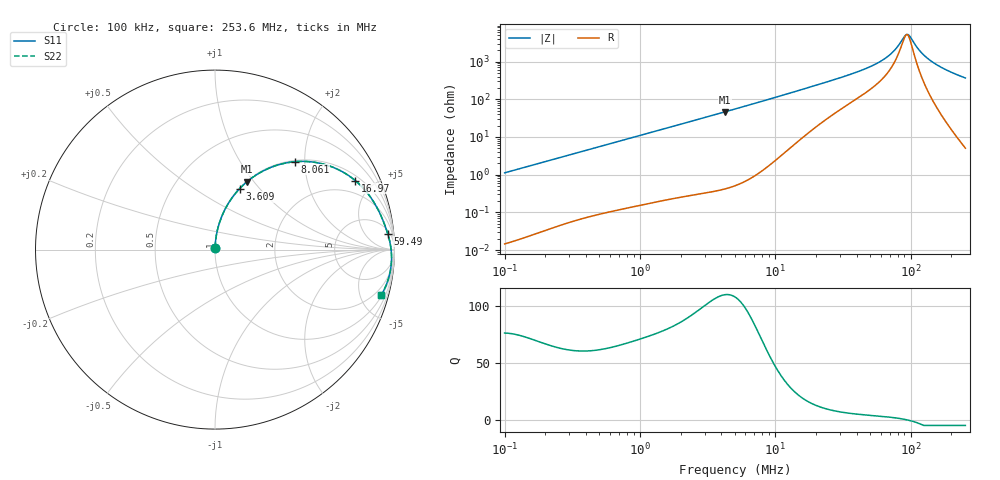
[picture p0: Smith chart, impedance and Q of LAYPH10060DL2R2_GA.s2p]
! LAYPH10060DL2R2_GA  S-PARAMETER MODEL  ( General Type )
! Model Generated by TAIYO YUDEN Corporation (http://www.ty-top.com)
! Version 3.0
! TAIYO YUDEN Control No. 180828NI43SB-FBB
! Copyright(c) 2017 TAIYO YUDEN CO.,LTD. All Rights Reserved.
! Product Description (link to TY-COMPAS)
! https://ds.yuden.co.jp/TYCOMPAS/or/detail?pn=LAYPH10060DL2R2NGA&u=M
! Products Name : Inductors
! Characteristics :
!  Inductance : 2.2 uH , SRF(min) : -Hz , DC Resistance(max) : 0.009 Ohm
!  Rated Current : Saturation :7.5 A , Temp Rise : 5.2 A (25 degC)
!  Case Size : 10.1 x 10.0 / 0.398 x 0.394 [mm/inch] , Thickness : 6 / 0.236 [mm/inch]
!  (Conditions: Temperature = 25 degC , DC Bias Current/Voltage = 0A / 0V)
! External Node Assignments :
!  1  o---GGG---o  2
! GND o---------o GND
! Frequency Range : 0.1MHz  -  253.640152MHz  [ 402 STEP ]
# MHz S RI R 50
! Freq[MHz].  S11 Real  S11 Imag  S21 Real  S21 Imag  S12 Real  S12 Imag  S22 Real  S22 Imag
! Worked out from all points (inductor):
!   401 points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, 100 kHz to 253.6 MHz, reference 50 ohm
!   read as one part in series: L = 1.78 uH near 104 kHz
!   highest Q = 110 at 4.222 MHz (marker M1), where L = 1.74 uH
!   self-resonance near 93.36 MHz
!   S11 on the Smith chart (normalised r, x): 100 kHz: 1.00, +0.02; 3.609 MHz: 1.01, +0.79; 8.061 MHz: 1.03, +1.79; 16.97 MHz: 1.23, +3.93; 59.49 MHz: 7, +19; 253.6 MHz: 1.10, -7.33
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0.1  0.000272 0.0112  0.9997 -0.0112  0.9997 -0.0112  0.000272 0.0112
0.371712  0.00237 0.0411  0.9976 -0.0411  0.9976 -0.0411  0.00237 0.0411
1.381698  0.0241 0.1471  0.9759 -0.1471  0.9759 -0.1471  0.0241 0.1471
2.345296  0.0637 0.2388  0.9363 -0.2388  0.9363 -0.2388  0.0637 0.2388
3.609356  0.1365 0.3387  0.8635 -0.3387  0.8635 -0.3387  0.1365 0.3387
4.22196  0.1776 0.3776  0.8224 -0.3776  0.8224 -0.3776  0.1776 0.3776
5.03627  0.2352 0.4195  0.7648 -0.4195  0.7648 -0.4195  0.2352 0.4195
8.060502  0.4448 0.4897  0.5552 -0.4897  0.5552 -0.4897  0.4448 0.4897
11.24712  0.6134 0.4738  0.3866 -0.4738  0.3866 -0.4738  0.6134 0.4738
16.97316  0.7815 0.3846  0.2185 -0.3846  0.2185 -0.3846  0.7815 0.3846
18.72042  0.8109 0.3579  0.1891 -0.3579  0.1891 -0.3579  0.8109 0.3579
38.655  0.9307 0.1752  0.0693 -0.1752  0.0693 -0.1752  0.9307 0.1752
59.48914  0.9621 0.0892  0.0379 -0.0892  0.0379 -0.0892  0.9621 0.0892
69.58603  0.9704 0.059  0.0296 -0.059  0.0296 -0.059  0.9704 0.059
78.26819  0.9756 0.0359  0.0244 -0.0359  0.0244 -0.0359  0.9756 0.0359
89.77577  0.9802 0.00818  0.0198 -0.00818  0.0198 -0.00818  0.9802 0.00818
95.21179  0.9816 -0.00406  0.0184 0.00406  0.0184 0.00406  0.9816 -0.00406
99.01747  0.9824 -0.0124  0.0176 0.0124  0.0176 0.0124  0.9824 -0.0124
118.1155  0.9837 -0.0512  0.0163 0.0512  0.0163 0.0512  0.9837 -0.0512
140.897  0.9808 -0.0927  0.0192 0.0927  0.0192 0.0927  0.9808 -0.0927
181.7769  0.9674 -0.1579  0.0326 0.1579  0.0326 0.1579  0.9674 -0.1579
253.6402  0.9276 -0.2523  0.0724 0.2523  0.0724 0.2523  0.9276 -0.2523
